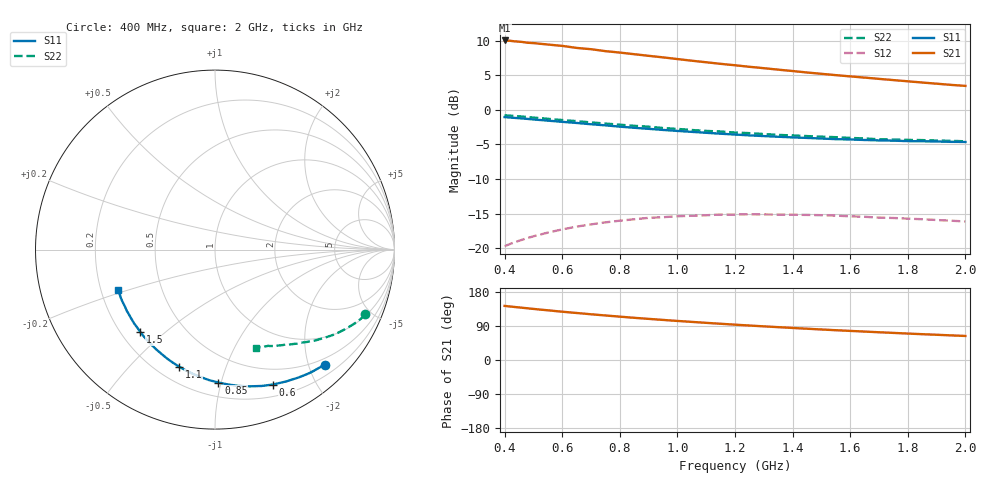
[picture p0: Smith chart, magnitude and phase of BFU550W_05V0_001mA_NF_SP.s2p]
! Filename:  P:\Prog\Test\Noise\ATS_data\Testdata_Net\06 Compressed Noise after Statistics\BFU550W_APM2013_11_D05_05p0V_001mA_NF_CM01_D.sf
! Date/Time: Tue 26/Mar/2013 16:25:20
! BFU550W_APM2013_11_D05_05p0V_1to35mA_NF_CM01_Bias1_R.sf
! Noise Parameter Data File
! BFU550W_APM2013_11_D05_05p0V_1to35mA_NF_CM01
! Date/time: Mon Mar 25 13:26:50 2013
! freq range =  0.4000 to  2.0000 GHz, 37 points
! bias range =  0.9950 to 35.0050 mA, 9 points
! bias supplies used: 1 1 0 0 0 0
! VAR bias_mode= 1  ! Specify V_out, I_out
! VAR bias_var = 1  ! Bias variable = I_out
! VAR V_out= 5.001000
! VAR I_out= 0.995000
! VAR V_in= 0.775700
! VAR I_in= 0.010001
! Device data file deembeded for feedlines and parallel
! Original file: \06 Compressed Noise after Statistics\BFU550W_APM2013_11_D05_05p0V_001mA_NF_CM01_R.sf
! Feed-files: PR019V01_070313_Feed1.s2p, PR019V01_070313_Feed2.s2p
! Parallel-file: PR019V01_070313_Par.s2p
# MHz S MA R 50
!  Freq-MHz  S11-mag  S11-arg  S21-mag  S21-arg  S12-mag  S12-arg  S22-mag  S22-arg
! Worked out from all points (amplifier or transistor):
!   37 points, 400 MHz to 2 GHz, reference 50 ohm
!   highest |S21| = 10.0 dB at 400 MHz (marker M1)
!   |S21| within 3 dB of that: start of sweep to 1.067 GHz
!   unconditionally stable (mu >= 1): nowhere
!   at 500 MHz: K = 0.20, MSG = 14.0 dB, |S12| = -18.3 dB
!   at 1.1 GHz: K = 0.42, MSG = 11.0 dB, |S12| = -15.2 dB
!   at 2 GHz: K = 0.81, MSG = 9.8 dB, |S12| = -16.1 dB
!   lowest NFmin = 0.48 dB at 420 MHz
!   S11 on the Smith chart (normalised r, x): 400 MHz: 0.39, -2.28; 600 MHz: 0.32, -1.47; 850 MHz: 0.30, -0.98; 1.1 GHz: 0.29, -0.70; 1.5 GHz: 0.28, -0.42; 2 GHz: 0.27, -0.19
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400  0.8852 -46.4  3.165 142.8  0.1035 61.3  0.9125 -23.3
420  0.878 -48.5  3.147 141.1  0.1076 60.1  0.9063 -24.3
440  0.8721 -50.6  3.117 139.5  0.1114 58.9  0.9001 -25.3
480  0.8585 -54.7  3.046 136.4  0.1185 56.6  0.8859 -27.2
500  0.8512 -56.8  3.029 134.8  0.122 55.4  0.8787 -28.0
600  0.8181 -66.7  2.892 127.5  0.1367 50.2  0.8428 -32.2
650  0.8029 -71.1  2.796 124.1  0.1432 47.9  0.8277 -34.0
700  0.7857 -75.8  2.737 120.7  0.1486 45.6  0.8102 -36.0
750  0.7714 -80.1  2.649 117.5  0.1538 43.6  0.7951 -37.6
800  0.7551 -84.4  2.588 114.4  0.1581 41.5  0.7798 -39.3
850  0.7408 -88.6  2.518 111.3  0.1619 39.6  0.7653 -40.8
950  0.7149 -96.3  2.389 105.8  0.1675 36.2  0.7379 -43.8
1000  0.7033 -100.1  2.323 103.1  0.1702 34.6  0.7274 -45.0
1100  0.6818 -107.2  2.202 98.0  0.1731 31.9  0.7032 -47.6
1200  0.6624 -113.9  2.096 93.2  0.175 29.4  0.6846 -50.1
1250  0.653 -117.2  2.042 91.0  0.1761 28.2  0.6779 -51.1
1350  0.6385 -123.4  1.948 86.7  0.175 26.5  0.6584 -53.5
1500  0.6198 -132.1  1.818 80.5  0.1732 24.1  0.6393 -56.8
1600  0.61 -137.6  1.742 76.8  0.1701 23.1  0.6261 -59.1
1750  0.5981 -145.3  1.637 71.5  0.1654 22.5  0.6098 -62.0
1850  0.5922 -150.1  1.573 68.1  0.162 22.3  0.6038 -64.1
2000  0.5853 -157.1  1.487 63.4  0.156 23.1  0.5919 -67.2
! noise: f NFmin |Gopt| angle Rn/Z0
400  0.4964  0.661  30.66  0.2979
460  0.511  0.6522  35.49  0.3174
600  0.5696  0.6696  44.29  0.3189
800  0.6298  0.6467  58.87  0.2665
1000  0.7929  0.6715  71.87  0.2816
1200  0.7793  0.6668  87.31  0.2316
1400  0.8275  0.6934  101.4  0.1684
1600  0.7328  0.6036  119.3  0.1179
1800  0.9402  0.6964  130.3  0.097
2000  1.021  0.7045  140.5  0.0788
